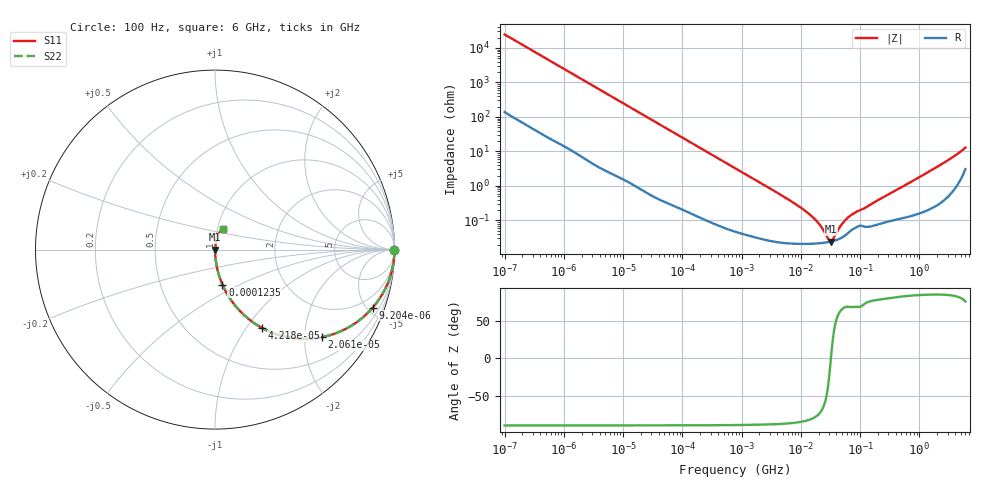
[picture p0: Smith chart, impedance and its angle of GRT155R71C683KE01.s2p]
!Murata Part Number: GRT155R71C683KE01
!These Parameters are Measured in Series Mode Connection
!Data Generated on Jun 19, 2026
!  o--ll--o
!Port1  Port2
!  o------o
!Operation Temp=25[degC], DC Bias Voltage=0[V]
!Freq. Start=100[Hz] Stop=6[GHz] 401[Steps]
# Hz S RI R 50
!Freq.(Hz) S11(Real) S11(Imag) S21(Real) S21(Imag) S12(Real) S12(Imag) S22(Real) S22(Imag)
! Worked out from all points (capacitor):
!   401 points, 100 Hz to 6 GHz, reference 50 ohm
!   read as one part in series: C = 64.7 nF near 109 Hz
!   lowest |Z| = 24.4 mohm at 31.85 MHz (marker M1)
!   series resonance near 32.2 MHz, so ESL is about 380 pH
!   S11 on the Smith chart (normalised r, x): 100 Hz: open; 9.204 kHz: 1.03, -5.43; 20.61 kHz: 1.02, -2.43; 42.18 kHz: 1.01, -1.19; 123.5 kHz: 1.00, -0.41; 6 GHz: 1.06, +0.25
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100  1 -0.00407  3.94e-05 0.00407  3.94e-05 0.00407  1 -0.00407
2008  0.9931 -0.0802  0.00694 0.0802  0.00694 0.0802  0.9931 -0.0802
4918  0.9615 -0.1896  0.0385 0.1896  0.0385 0.1896  0.9615 -0.1896
9204  0.8789 -0.3232  0.1211 0.3232  0.1211 0.3232  0.8789 -0.3232
20606  0.5959 -0.4876  0.4041 0.4876  0.4041 0.4876  0.5959 -0.4876
40335  0.2806 -0.446  0.7194 0.446  0.7194 0.446  0.2806 -0.446
42182  0.2631 -0.437  0.7369 0.437  0.7369 0.437  0.2631 -0.437
69028  0.1191 -0.3202  0.8809 0.3202  0.8809 0.3202  0.1191 -0.3202
123542  0.0416 -0.1954  0.9584 0.1954  0.9584 0.1954  0.0416 -0.1954
276587  0.00923 -0.0907  0.9908 0.0907  0.9908 0.0907  0.00923 -0.0907
774597  0.00155 -0.0328  0.9985 0.0328  0.9985 0.0328  0.00155 -0.0328
6353432  0.000229 -0.0039  0.9998 0.0039  0.9998 0.0039  0.000229 -0.0039
1.555665e7  0.000212 -0.00127  0.9998 0.00127  0.9998 0.00127  0.000212 -0.00127
2.035112e7  0.000217 -0.00076  0.9998 0.00076  0.9998 0.00076  0.000217 -0.00076
2.911731e7  0.000235 -0.000161  0.9998 0.000161  0.9998 0.000161  0.000235 -0.000161
3.184506e7  0.000243 -1.76e-05  0.9998 1.76e-05  0.9998 1.76e-05  0.000243 -1.76e-05
3.482834e7  0.000252 0.000126  0.9997 -0.000126  0.9997 -0.000126  0.000252 0.000126
4.983056e7  0.000321 0.000723  0.9997 -0.000723  0.9997 -0.000723  0.000321 0.000723
6.518806e7  0.000459 0.0012  0.9995 -0.0012  0.9995 -0.0012  0.000459 0.0012
3.124326e8  0.000975 0.00578  0.999 -0.00578  0.999 -0.00578  0.000975 0.00578
2.048624e9  0.00412 0.0362  0.9959 -0.0362  0.9959 -0.0362  0.00412 0.0362
6e9  0.0438 0.1159  0.9562 -0.1159  0.9562 -0.1159  0.0438 0.1159
